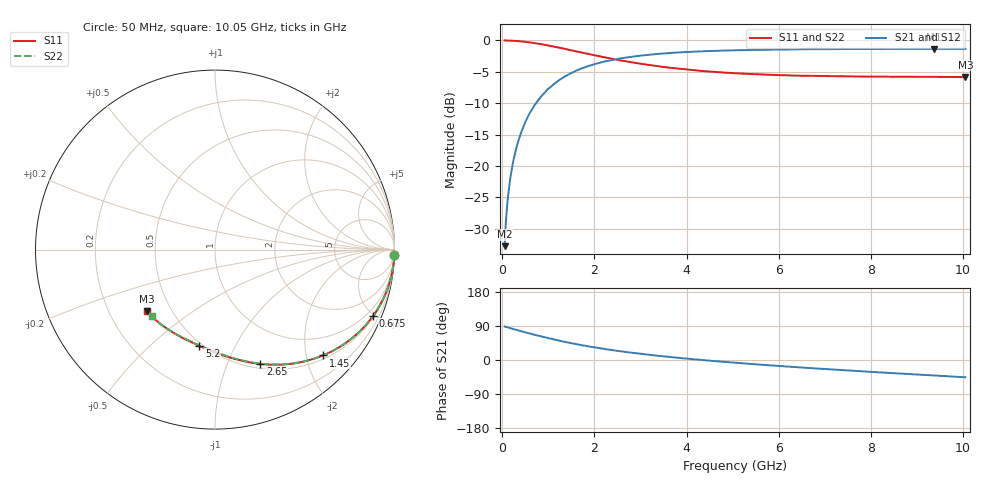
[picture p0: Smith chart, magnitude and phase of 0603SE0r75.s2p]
! AVX Thin Film Operation		Date: August 2001
! Description: Accu-P® Series, Thin Film, SMD, RF Capacitor
! Part Number: 06035J0R75ABT
! 50 MHz  -  10.05 GHz
! Serial Measurements
# mhz S db R 50
!	S11		S21		S12		S22
!	dB	Phase	dB	Phase	dB	Phase	dB	Phase
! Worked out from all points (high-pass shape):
!   401 points, 50 MHz to 10.05 GHz, reference 50 ohm
!   highest |S21| = -1.35 dB at 9.375 GHz (marker M1); lowest = -32.8 dB at 50 MHz (marker M2)
!   |S21| within 3 dB of the highest: 1.762 GHz to end of sweep
!   lowest |S11| = -5.8 dB at 10.05 GHz (marker M3), VSWR 3.09, Z = 18.3 - j17 ohm
!   |S11| at or under -10 dB: nowhere
!   |S22| runs from -5.8 to 0.0 dB; largest |S21 - S12| = 0
!   S11 on the Smith chart (normalised r, x): 50 MHz: 1, -66; 675 MHz: 0.58, -4.92; 1.45 GHz: 0.57, -2.33; 2.65 GHz: 0.55, -1.32; 5.2 GHz: 0.48, -0.73; 10.05 GHz: 0.37, -0.34
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50  -0.00 -1.7  -32.80 88.3  -32.80 88.3  -0.00 -1.7
75  -0.01 -2.6  -29.21 87.4  -29.21 87.4  -0.01 -2.6
125  -0.01 -4.3  -24.79 85.7  -24.79 85.7  -0.01 -4.3
150  -0.02 -5.2  -23.27 84.8  -23.27 84.8  -0.02 -5.2
200  -0.04 -6.9  -20.78 83.1  -20.78 83.1  -0.04 -6.9
275  -0.07 -9.5  -18.04 80.5  -18.04 80.5  -0.07 -9.5
350  -0.11 -12.0  -15.99 78.0  -15.99 78.0  -0.11 -12.0
450  -0.18 -15.3  -13.93 74.7  -13.93 74.7  -0.18 -15.3
675  -0.40 -22.7  -10.64 67.3  -10.64 67.3  -0.40 -22.7
1000  -0.81 -32.6  -7.68 57.4  -7.68 57.4  -0.81 -32.6
1450  -1.49 -44.5  -5.38 45.5  -5.38 45.5  -1.49 -44.4
1725  -1.93 -50.9  -4.46 39.1  -4.46 39.1  -1.93 -50.8
2175  -2.62 -60.0  -3.45 30.0  -3.45 30.0  -2.62 -59.9
2650  -3.29 -68.4  -2.76 21.6  -2.76 21.6  -3.29 -68.2
3400  -4.13 -79.2  -2.13 10.9  -2.13 10.9  -4.12 -78.8
4125  -4.73 -88.0  -1.80 2.2  -1.80 2.2  -4.73 -87.3
5050  -5.24 -97.7  -1.56 -7.3  -1.56 -7.3  -5.22 -96.6
5200  -5.29 -99.2  -1.54 -8.7  -1.54 -8.7  -5.28 -97.9
6725  -5.66 -112.9  -1.40 -21.7  -1.40 -21.7  -5.64 -110.0
8400  -5.78 -125.2  -1.36 -34.2  -1.36 -34.2  -5.76 -122.2
9375  -5.81 -132.6  -1.35 -41.0  -1.35 -41.0  -5.78 -128.6
10050  -5.83 -137.8  -1.35 -45.6  -1.35 -45.6  -5.80 -133.4
